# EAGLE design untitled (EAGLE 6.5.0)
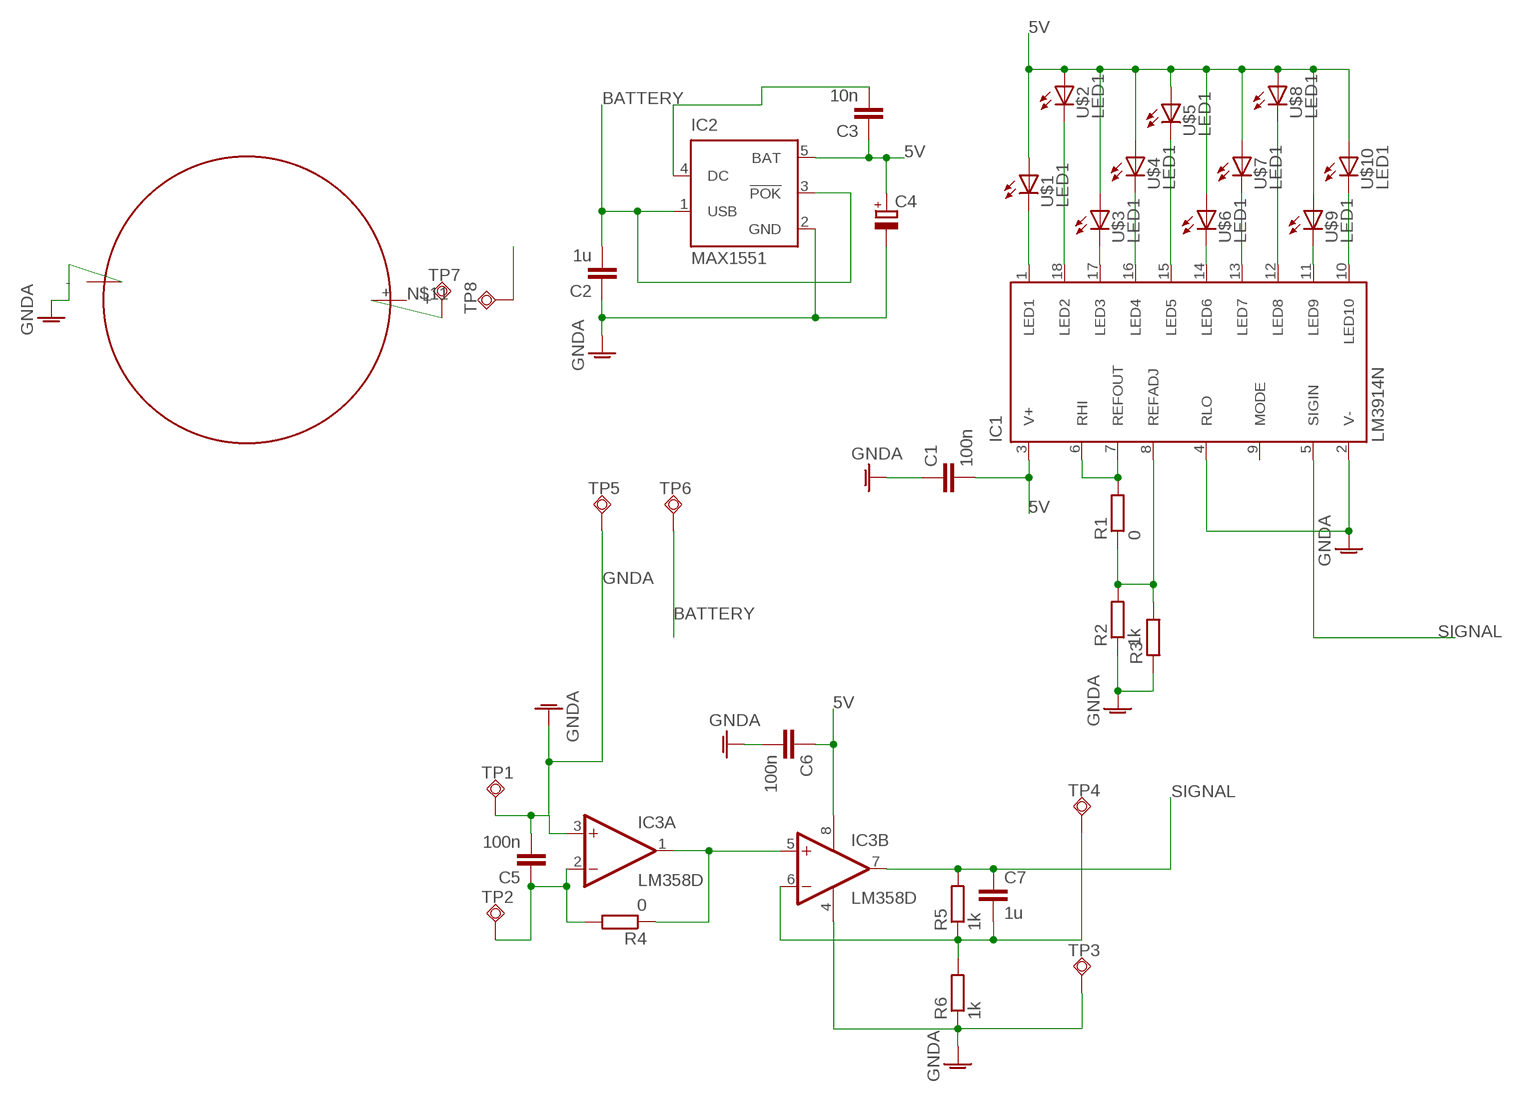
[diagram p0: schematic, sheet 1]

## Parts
C1  100n  C-EUC0805  [C0805]
C2  1u  C-EUC0805  [C0805]
C3  10n  C-EUC0805  [C0805]
C4  CPOL-EU150CLZ-0810  [150CLZ-0810]
C5  100n  C-EUC0805  [C0805]
C6  100n  C-EUC0805  [C0805]
C7  1u  C-EUC0805  [C0805]
IC1  LM3914N  [DIL18]
IC2  MAX1551  [SOT23-5L]
IC3  LM358D  [SO08]
R1  0  R-EU_R0805  [R0805]
R2  1k  R-EU_R0805  [R0805]
R3  R-EU_R0805  [R0805]
R4  0  R-EU_R0805  [R0805]
R5  1k  R-EU_R0805  [R0805]
R6  1k  R-EU_R0805  [R0805]
TP1  TPSQB2,54  [B2,54]
TP2  TPSQB2,54  [B2,54]
TP3  TPSQB2,54  [B2,54]
TP4  TPSQB2,54  [B2,54]
TP5  TPSQB2,54  [B2,54]
TP6  TPSQB2,54  [B2,54]
TP7  TPSQB2,54  [B2,54]
TP8  TPSQB2,54  [B2,54]
U$1  LED1  [LED1]
U$2  LED1  [LED1]
U$3  LED1  [LED1]
U$4  LED1  [LED1]
U$5  LED1  [LED1]
U$6  LED1  [LED1]
U$7  LED1  [LED1]
U$8  LED1  [LED1]
U$9  LED1  [LED1]
U$10  LED1  [LED1]
U$11  CR2032  [CR2023]

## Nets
5V: C1.2 C3.1 C4.+ C6.1 IC1.3(V+) IC2.5(BAT) IC3.8(P:V+) U$1.A U$2.A U$3.A U$4.A U$5.A U$6.A U$7.A U$8.A U$9.A U$10.A
BATTERY: C2.2 IC2.1(USB) IC2.3(!POK) TP6.TP TP8.TP
GNDA: C1.1 C2.1 C4.- C5.2 C6.2 IC1.2(V-) IC1.4(RLO) IC2.2(GND) IC3.3(A:+IN) IC3.4(P:V-) R2.1 R3.1 R6.1 TP1.TP TP3.TP TP5.TP U$11.-
N$1: IC1.1(LED1) U$1.K(C)
N$2: IC1.18(LED2) U$2.K(C)
N$3: IC1.17(LED3) U$3.K(C)
N$4: IC1.16(LED4) U$4.K(C)
N$5: IC1.15(LED5) U$5.K(C)
N$6: IC1.14(LED6) U$6.K(C)
N$7: IC1.13(LED7) U$7.K(C)
N$8: IC1.12(LED8) U$8.K(C)
N$9: IC1.11(LED9) U$9.K(C)
N$10: IC1.10(LED10) U$10.K(C)
N$11: TP7.TP U$11.+
N$12: C3.2 IC2.4(DC)
N$13: C5.1 IC3.2(A:-IN) R4.2 TP2.TP
N$14: IC1.8(REFADJ) R1.1 R2.2 R3.2
N$15: IC1.6(RHI) IC1.7(REFOUT) R1.2
N$16: IC3.1(A:OUT) IC3.5(B:+IN) R4.1
N$18: C7.2 IC3.6(B:-IN) R5.1 R6.2 TP4.TP
SIGNAL: C7.1 IC1.5(SIGIN) IC3.7(B:OUT) R5.2
Unconnected: IC1.9(MODE)

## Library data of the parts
C1-C3 C5-C7 = rcl:C-EU: CAPACITOR, European symbol
C4 = rcl:CPOL-EU: POLARIZED CAPACITOR, European symbol
IC1 = national-semiconductor:LM391: Dot/Bar Display Driver Source: Data sheet LM3915 Data sheet LM3914
IC2 = maxim:MAX1551: Dual-Input USB/AC Adapter 1-Cell Li+ Battery Chargers Source: http://www.maxim-ic.com .. MAX1551-MAX1555.pdf; MF: MAXIM; MPN: MAX1551EZK-T; OC_FARNELL: 1628221; OC_NEWARK: 88H0599
IC3 = linear:LM358: OP AMP also LM158; LM258; LM2904 Source: http://cache.national.com/ds/LM/LM158.pdf
R1-R6 = rcl:R-EU_: RESISTOR, European symbol
TP1-TP8 = testpad:TPSQ: Test pad
U$1-U$10 = led:LED1
U$11 = eigeneBauteile:CR2032

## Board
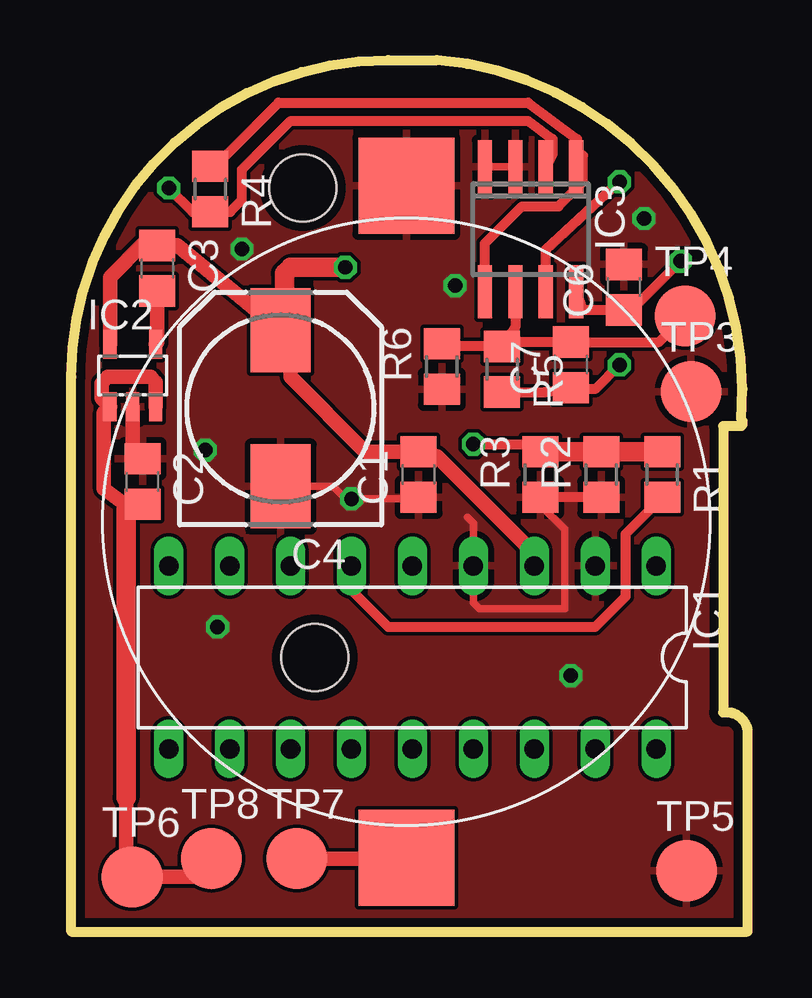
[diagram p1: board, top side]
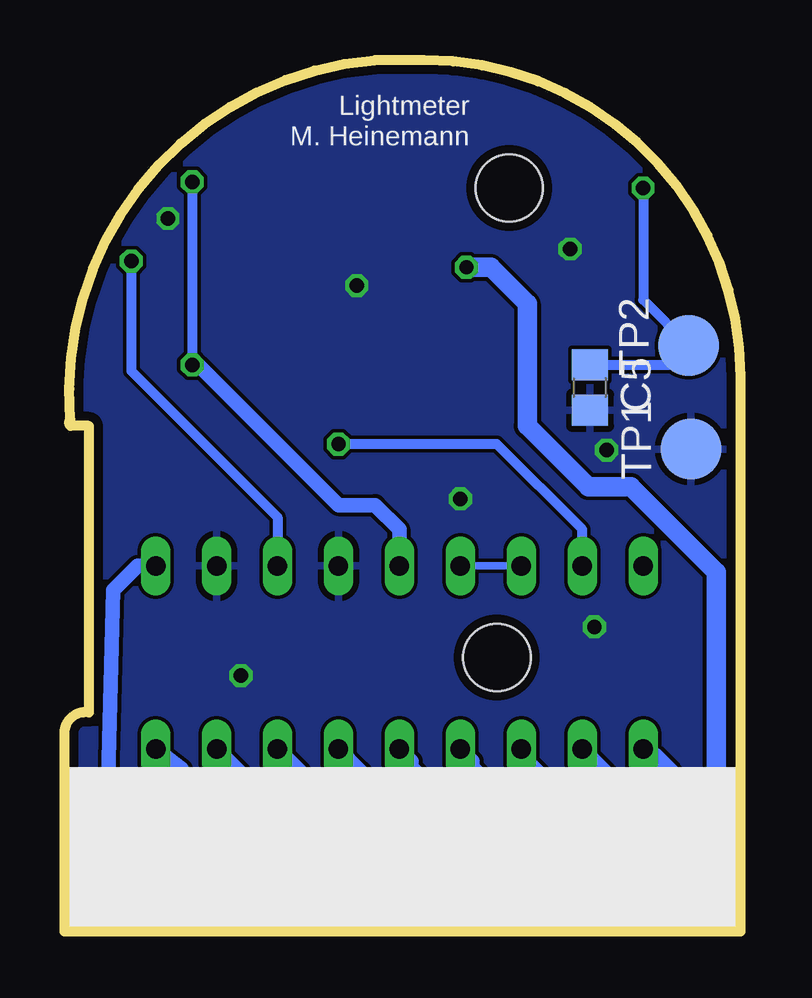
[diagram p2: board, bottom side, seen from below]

Size 28.19 x 36.32 mm. Coordinates in mm from the lower left corner, seen from the top.
Outline: 0,0 28.19,0 28.19,8.38 arc90 27.18,9.14 27.18,21.08 27.94,21.08 arc90 27.94,21.34 arc90 15.24,36.32 13.21,36.32 arc90 0,23.11 0,0
Copper layers (1*16): Top 0.0356mm / dielectric 1.5011mm / Bottom 0.0356mm
Design rules "LaenPCBOrder": minimum track width 6mil, minimum drill 13mil, track to track 6mil, track to pad 6mil, pad to pad 6mil, via to via 6mil, smd to smd 6mil, copper to edge 15mil, drill to drill 6mil, minimum pad ring 7mil, minimum via ring 7mil, stop-mask expansion 3mil, vias tented up to drill 0mil, thermal gap 10mil
Holes 2.8 mm at 9.65,30.99 10.16,11.43

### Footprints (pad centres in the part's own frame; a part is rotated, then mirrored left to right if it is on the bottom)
C0805 = smd 1.3 x 1.5: 1 -0.95,0; 2 0.95,0
150CLZ-0810 = smd 3.5 x 2.5: + 3.25,0; - -3.25,0
DIL18 = drill 0.813 long: 1 -10.16,-3.81; 2 -7.62,-3.81; 3 -5.08,-3.81; 4 -2.54,-3.81; 5 0,-3.81; 6 2.54,-3.81; 7 5.08,-3.81; 8 7.62,-3.81; 9 10.16,-3.81; 10 10.16,3.81; 11 7.62,3.81; 12 5.08,3.81; 13 2.54,3.81; 14 0,3.81; 15 -2.54,3.81; 16 -5.08,3.81; 17 -7.62,3.81; 18 -10.16,3.81
SOT23-5L = smd 0.55 x 1.2: 1 -0.95,-1.3; 2 0,-1.3; 3 0.95,-1.3; 4 0.95,1.3; 5 -0.95,1.3
SO08 = smd 0.6 x 2.2: 1 -1.905,-2.6; 2 -0.635,-2.6; 3 0.635,-2.6; 4 1.905,-2.6; 5 1.905,2.6; 6 0.635,2.6; 7 -0.635,2.6; 8 -1.905,2.6
R0805 = smd 1.3 x 1.5: 1 -0.95,0; 2 0.95,0
B2,54 = smd 2.54 x 2.54: TP 0,0
LED1 = smd 2.2 x 2.2: A 0,3.73; K 0,0.635
CR2023 = smd 4 x 4: + 0,-2; - 0,26

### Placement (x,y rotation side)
C1  14.48,19.05 90 top
C2  2.97,18.76 270 top
C3  3.59,27.65 270 top
C4  8.73,21.8 90 top
C5  6.28,22.68 270 bottom
C6  23.04,26.85 90 top
C7  20.83,23.62 90 top
IC1  14.22,11.43 180 top
IC2  2.56,23.18 0 top
IC3  19.15,29.27 180 top
R1  24.64,19.05 270 top
R2  22.1,19.05 90 top
R3  19.56,19.05 90 top
R4  5.8,30.95 270 top
R5  17.96,23.44 270 top
R6  15.45,23.55 90 top
TP1  2.07,20.11 90 bottom
TP2  2.16,24.42 90 bottom
TP3  25.84,22.5 0 top
TP4  25.58,25.65 0 top
TP5  25.65,2.54 0 top
TP6  2.54,2.29 0 top
TP7  9.4,3.05 0 top
TP8  5.84,3.05 0 top
U$1  25.79,5.35 180 bottom
U$2  23.29,5.35 180 bottom
U$3  20.8,5.35 180 bottom
U$4  18.31,5.35 180 bottom
U$5  15.82,5.35 180 bottom
U$6  12.82,5.35 180 bottom
U$7  10.33,5.35 180 bottom
U$8  7.83,5.35 180 bottom
U$9  5.34,5.35 180 bottom
U$10  2.85,5.35 180 bottom
U$11  13.97,5.08 0 top

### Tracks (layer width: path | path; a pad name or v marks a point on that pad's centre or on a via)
5V  (via drill 0.6 pad 0.81)
  Top 0.406: IC3.8 21.34,25.91 C6.1 23.3,26.16 23.62,26.16 v25.4,27.94
  Top 0.61: IC2.5 1.61,27.27 3.05,28.7 3.48,28.7 C3.1 4.42,28.6 C4.+ 9.14,24.64 9.14,23.11 12.26,20 C1.2 15.17,19.81 15.24,19.81 19.3,15.75 IC1.3
  Top 0.813: v11.43,27.69 9.14,27.69 8.89,27.43 8.89,25.22 C4.+
  Bottom 0.406: v25.4,27.94 25.4,23.37 19.3,17.27 IC1.3
  Bottom 0.813: U$4.A 1.68,1.62 1.02,2.29 1.02,14.99 4.57,18.54 6.35,18.54 8.89,21.08 8.89,26.16 10.41,27.69 v11.43,27.69
  Bottom 1.016: U$10.A U$9.A U$8.A U$7.A U$6.A U$5.A | U$5.A 15.4,1.62 15.75,1.27 15.66,1.27 U$5.A | U$5.A U$4.A U$3.A U$2.A U$1.A
BATTERY
  Top 0.61: IC2.3 3.51,22.9 3.3,23.11 1.52,23.11 1.27,22.86 1.27,22.22 IC2.1 1.36,21.62 1.36,18.45 2.29,17.78 2.94,17.78 C2.2 | 2.29,5.59 2.29,2.54 TP6.TP 5.08,2.29 TP8.TP
  Top 0.813: 2.29,17.78 2.29,5.59
GNDA  (via drill 0.6 pad 0.81)
  Top 0.305: IC3.4 IC3.3 | 16.51,17.27 16.76,17.02 IC1.4 16.76,13.72 17.02,13.46 20.57,13.46 20.57,16.76 19.56,17.78 R3.1 | C4.- 10.91,18.55 11.43,18.03 14.41,18.03 C1.1
  Top 0.406: R2.1 R3.1 | 14.79,18.55 C1.1 14.67,18.1
  Top 0.61: IC2.2 2.56,20.11 C2.1
  other vias: 11.68,18.03 6.1,12.7 20.83,10.67 7.11,28.45 5.59,20.07 16,26.92 23.88,29.72
  pour Top: 0.25,0 27.69,0 27.69,20.83 27.69,25.15 arc90 14.99,37.85 11.68,37.85 arc90 0,26.16 0,0.25 arc90
  pour Bottom: 0,0 27.69,0 27.69,25.65 arc90 17.27,36.07 11.43,36.07 arc90 0.25,24.89
N$1
  Bottom 0.305: 25.65,5.61 U$1.K
  Bottom 0.61: IC1.1 25.15,15.24 26.16,14.22 26.42,4.84 U$1.K
N$2
  Bottom 0.61: U$2.K 23.29,6.78 IC1.18
N$3
  Bottom 0.61: U$3.K 20.8,6.58 IC1.17
N$4
  Bottom 0.61: U$4.K 18.31,6.63 IC1.16
N$5
  Bottom 0.61: U$5.K 15.82,6.67 IC1.15
N$6
  Bottom 0.61: U$6.K 12.82,5.96 13.72,6.86 13.72,7.11 IC1.14
N$7
  Bottom 0.61: U$7.K 9.82,5.5 11.18,6.86 11.18,7.11 IC1.13
N$8
  Bottom 0.61: U$8.K 7.33,5.55 8.89,7.11 8.89,7.37 IC1.12
N$9
  Bottom 0.61: U$9.K 4.58,5.6 IC1.11
N$10
  Bottom 0.61: U$10.K 2.85,6.66 3.56,7.37 3.81,7.37 IC1.10
N$11
  Top 0.61: TP7.TP 13.94,3.05 U$11.+
N$12
  Top 0.61: C3.2 3.59,24.55 IC2.4
N$13  (via drill 0.6)
  Top 0.406: v4.06,30.99 5.05,30 R4.2 6.63,30 7.11,30.48 7.11,31.75 9.14,33.78 19.05,33.78 20.07,33.02 20.07,32.4 IC3.2
  Bottom 0.406: C5.1 2.96,23.63 TP2.TP 4.06,26.32 v4.06,30.99
N$14  (via drill 0.6)
  Top 0.406: v16.76,20.32 19.24,20.32 R3.2
  Top 0.813: R1.1 R2.2 R3.2
  Bottom 0.406: IC1.8 6.6,16.76 10.16,20.32 v16.76,20.32
N$15
  Top 0.406: IC1.6 11.68,14.22 13.21,12.7 21.84,12.7 23.11,13.97 23.11,16.58 R1.2
  Bottom 0.305: IC1.6 IC1.7
N$16
  Top 0.406: IC3.5 17.25,28.68 18.8,30.23 20.32,30.23 21.34,31.24 21.34,32.35 IC3.1 21.08,32.4 21.08,33.02 19.05,34.54 8.64,34.54 6.24,32.15 6.24,31.9 R4.1
N$18
  Top 0.406: R5.1 15.06,24.39 R6.2 | R5.1 17.78,24.57 C7.2 24.51,24.57 TP4.TP | IC3.6 18.52,25.2 R5.1
SIGNAL  (via drill 0.6, 0.6 pad 0.81)
  Top 0.406: R5.2 19.74,22.49 C7.1 20.25,22.61 21.84,22.61 v22.86,23.62 | IC3.7 19.79,28.42 v22.86,31.24
  Bottom 0.406: v22.86,31.24 v22.86,23.62
  Bottom 0.61: v22.86,23.62 22.61,23.62 16.76,17.78 15.24,17.78 14.22,16.76 IC1.5

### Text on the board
bNames: Lightmeter | M. Heinemann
